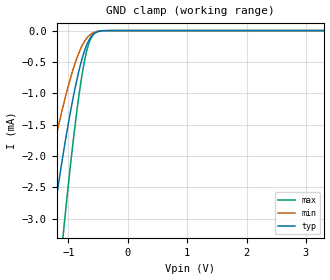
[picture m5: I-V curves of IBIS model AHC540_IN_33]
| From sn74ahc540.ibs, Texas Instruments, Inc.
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[Model]   AHC540_IN_33
Model_type  Input
Vinl = 0.9
Vinh = 2.1
| variable   typ   min   max
C_comp   0.58pF   0.53pF   0.65pF
[Temperature Range]   40   100   -40
| Ambient temperature   25   85   -40
[Voltage range]   3.3   3   3.6
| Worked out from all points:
|   GND clamp passes 1 mA (typ) near -0.91 V on its own axis
[GND Clamp]
| AHC540_IN_33
|   Voltage   I(typ)   I(min)   I(max)
-5V       -39.52mA   -26.01mA   -50.56mA
-1.55V    -5.112mA   -3.269mA   -8.043mA
-1.5V     -4.735mA   -3.021mA   -7.495mA
-1.295V   -3.277mA   -2.063mA   -5.315mA
-1.245V   -2.945mA   -1.844mA   -4.802mA
-1.08V    -1.923mA   -1.171mA   -3.185mA
-910mV    -1.022mA   -586uA     -1.69mA
-785mV    -502.6uA   -271.2uA   -792.7uA
-680mV    -204uA     -109.1uA   -284uA
-630mV    -114.1uA   -63.52uA   -144.4uA
-555mV    -38.56uA   -23.82uA   -40.51uA
3.3V      3.885nA    645.3pA    18.64nA
